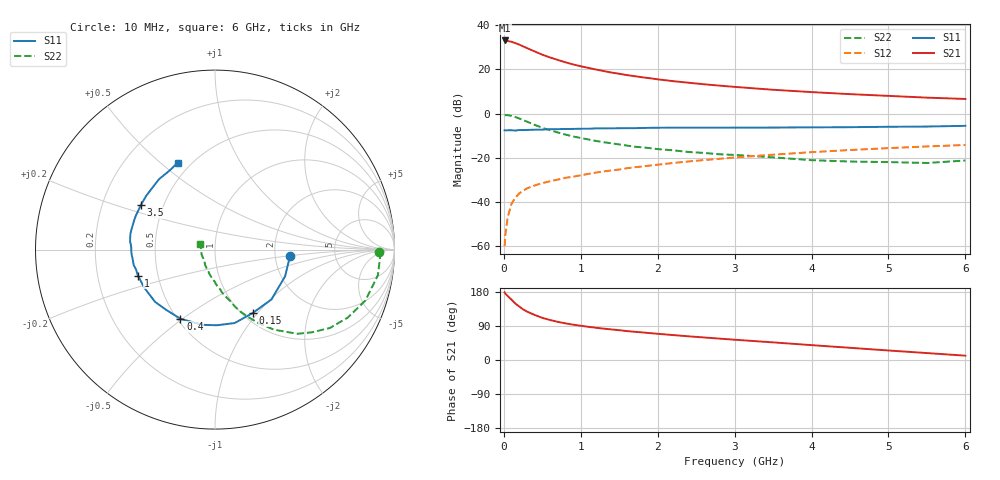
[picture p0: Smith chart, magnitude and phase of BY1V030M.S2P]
! SIEMENS Small Signal Semiconductors
! BFY420
! Si NPN RF SIEGET Grounded Emitter Transistor in MICRO-X
! VCE = 1 V  IC = 30 mA
! Common Emitter S-Parameters:  October  1996
# GHz  S  MA  R  50
!  f  S11  S21  S12  S22
! GHz  MAG  ANG  MAG  ANG  MAG  ANG  MAG  ANG
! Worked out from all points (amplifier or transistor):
!   36 points, 10 MHz to 6 GHz, reference 50 ohm
!   highest |S21| = 33.1 dB at 10 MHz (marker M1)
!   |S21| within 3 dB of that: start of sweep to 271.7 MHz
!   unconditionally stable (mu >= 1): start of sweep to 15.81 MHz; 1.396 GHz to end of sweep
!   at 250 MHz: K = 0.39, MSG = 32.6 dB, |S12| = -34.9 dB
!   at 1.4 GHz: K = 1.00, MAG = 21.9 dB, |S12| = -25.7 dB
!   at 6 GHz: K = 1.09, MAG = 8.5 dB, |S12| = -14.2 dB
!   S11 on the Smith chart (normalised r, x): 10 MHz: 2.41, -0.22; 150 MHz: 1.11, -0.94; 400 MHz: 0.52, -0.49; 1 GHz: 0.38, -0.14; 3.5 GHz: 0.37, +0.24; 6 GHz: 0.43, +0.57
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0.01  0.4181 -5.2  44.95 178.5  0.001 97.8  0.912 -0.8
0.02  0.4159 -9.0  44.82 175.1  0.0018 86.9  0.9204 -2.8
0.05  0.418 -20.9  43.59 168.9  0.0045 83.6  0.9188 -8.9
0.1  0.4195 -41.5  42.02 159.0  0.0091 75.0  0.8847 -18.7
0.15  0.411 -59.3  39.05 148.8  0.0125 70.1  0.8311 -27.1
0.2  0.4236 -75.0  36.27 141.2  0.0156 66.7  0.775 -34.3
0.25  0.4217 -88.6  33.09 133.7  0.018 62.9  0.7096 -40.5
0.3  0.425 -99.5  30.24 127.9  0.0202 61.8  0.6565 -45.6
0.4  0.4309 -116.5  25.39 118.9  0.0236 58.7  0.5544 -53.6
0.5  0.4322 -129.2  21.42 111.2  0.0266 56.7  0.4765 -59.4
0.6  0.4431 -138.9  18.57 105.6  0.0294 56.7  0.4184 -63.8
0.7  0.4428 -145.8  16.32 100.7  0.032 57.0  0.3733 -67.7
0.8  0.4478 -151.9  14.43 96.7  0.0351 56.2  0.3344 -70.9
1  0.4534 -161.3  11.73 90.4  0.0401 57.4  0.2797 -75.6
1.1  0.4537 -165.8  10.75 87.5  0.0432 57.6  0.2592 -78.6
1.4  0.4624 -174.2  8.437 80.7  0.0517 58.2  0.2123 -84.6
1.6  0.4669 -179.5  7.404 76.3  0.0579 57.5  0.1884 -89.1
2.2  0.4794 169.1  5.4 65.8  0.076 55.3  0.1475 -100.0
3.5  0.4817 148.9  3.446 46.5  0.1173 46.5  0.102 -122.7
4.5  0.4909 135.0  2.744 32.2  0.1496 37.3  0.082 -142.0
5.5  0.5079 119.9  2.288 18.3  0.1802 27.1  0.0761 179.7
6  0.527 113.2  2.135 11.4  0.1943 21.8  0.0866 160.7
